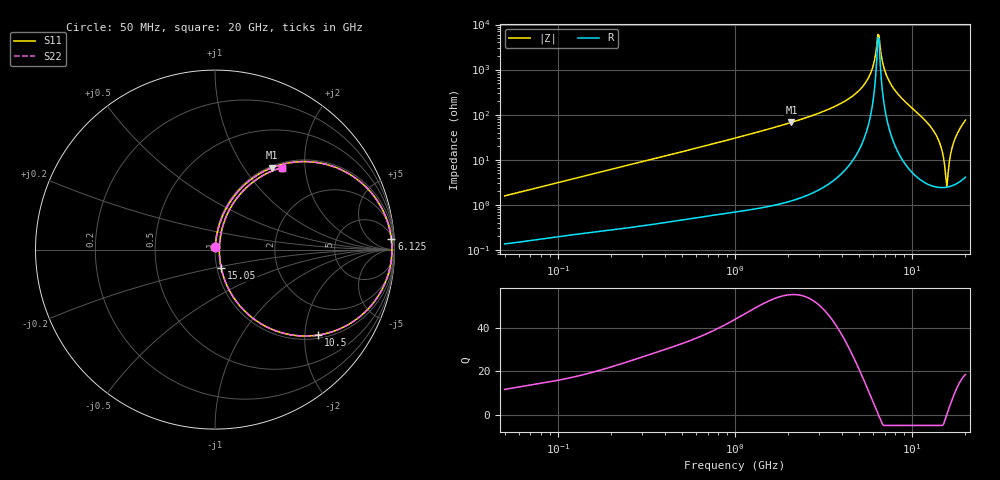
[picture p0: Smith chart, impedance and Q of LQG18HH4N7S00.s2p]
!Murata Part Number: LQG18HH4N7S00
!These Parameters are Measured in Series Mode Connection
!  o--[Z]--o
!Port1  Port2
!  o-------o
!Freq. Start=50[MHz] Stop=20[GHz], 401[Steps]
# Hz S RI R 50
!Freq.(Hz) S11(Real) S11(Imag) S21(Real) S21(Imag) S12(Real) S12(Imag) S22(Real) S22(Imag)
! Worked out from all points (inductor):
!   401 points, 50 MHz to 20 GHz, reference 50 ohm
!   read as one part in series: L = 4.97 nH near 51.52 MHz
!   highest Q = 55.2 at 2.083 GHz (marker M1), where L = 5.15 nH
!   self-resonance near 6.407 GHz
!   S11 on the Smith chart (normalised r, x): 50 MHz: 1.00, +0.03; 6.125 GHz: 8, +31; 10.5 GHz: 1.09, -2.34; 15.05 GHz: 1.05, -0.22; 20 GHz: 1.08, +1.51
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5e7  0.0016 0.0156  0.9984 -0.0156  0.9984 -0.0156  0.0016 0.0156
1.364002e8  0.00401 0.0414  0.996 -0.0414  0.996 -0.0414  0.00401 0.0414
3.721004e8  0.016 0.1095  0.984 -0.1095  0.984 -0.1095  0.016 0.1095
1e9  0.0885 0.2728  0.9115 -0.2728  0.9115 -0.2728  0.0885 0.2728
2.083303e9  0.3155 0.4557  0.6845 -0.4557  0.6845 -0.4557  0.3155 0.4557
2.728004e9  0.4763 0.49  0.5237 -0.49  0.5237 -0.49  0.4763 0.49
4.81993e9  0.8884 0.2947  0.1116 -0.2947  0.1116 -0.2947  0.8884 0.2947
5.598765e9  0.9604 0.1576  0.0396 -0.1576  0.0396 -0.1576  0.9604 0.1576
6.125241e9  0.9824 0.0601  0.0176 -0.0601  0.0176 -0.0601  0.9824 0.0601
6.311513e9  0.9852 0.0256  0.0148 -0.0256  0.0148 -0.0256  0.9852 0.0256
6.503449e9  0.9856 -0.00957  0.0144 0.00957  0.0144 0.00957  0.9856 -0.00957
7.009217e9  0.9749 -0.0997  0.0251 0.0997  0.0251 0.0997  0.9749 -0.0997
7.442007e9  0.9532 -0.1723  0.0468 0.1723  0.0468 0.1723  0.9532 -0.1723
8.516016e9  0.8574 -0.3263  0.1426 0.3263  0.1426 0.3263  0.8574 -0.3263
1.050288e10  0.5763 -0.476  0.4237 0.476  0.4237 0.476  0.5763 -0.476
1.334722e10  0.1602 -0.3373  0.8398 0.3373  0.8398 0.3373  0.1602 -0.3373
1.438523e10  0.0671 -0.2015  0.9329 0.2015  0.9329 0.2015  0.0671 -0.2015
1.504638e10  0.0344 -0.1024  0.9656 0.1024  0.9656 0.1024  0.0344 -0.1024
1.527346e10  0.0283 -0.0673  0.9717 0.0673  0.9717 0.0673  0.0283 -0.0673
1.573793e10  0.0241 0.00506  0.9759 -0.00506  0.9759 -0.00506  0.0241 0.00506
1.747767e10  0.0992 0.2542  0.9008 -0.2542  0.9008 -0.2542  0.0992 0.2542
2e10  0.3711 0.4567  0.6289 -0.4567  0.6289 -0.4567  0.3711 0.4567
